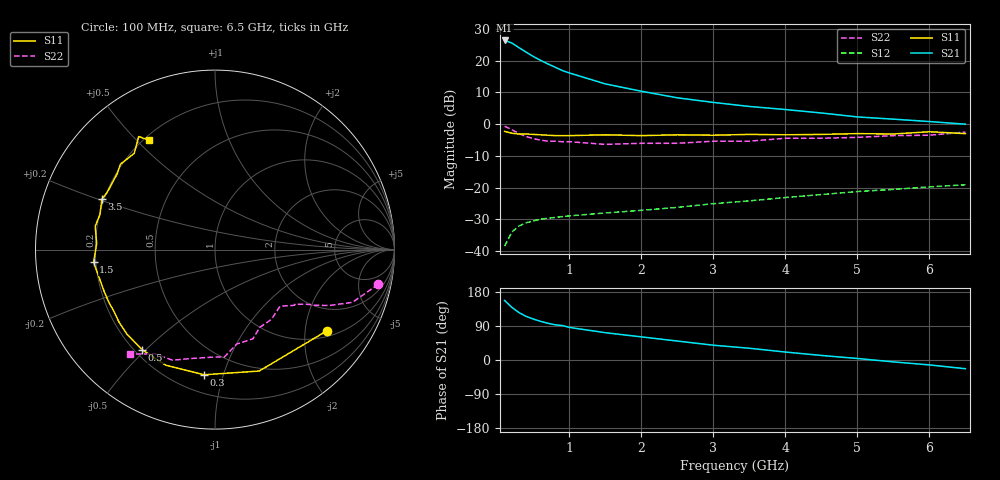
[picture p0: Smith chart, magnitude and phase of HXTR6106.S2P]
! HXTR-6106 Common Emitter
! Vce=15V  Ic=10mA
# ghz s ma r 50
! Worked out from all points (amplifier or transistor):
!   21 points, 100 MHz to 6.5 GHz, reference 50 ohm
!   highest |S21| = 26.4 dB at 100 MHz (marker M1)
!   |S21| within 3 dB of that: start of sweep to 351.1 MHz
!   unconditionally stable (mu >= 1): 1.454 GHz to 4.9 GHz
!   at 400 MHz: K = 0.38, MSG = 26.9 dB, |S12| = -31.1 dB
!   at 1.5 GHz: K = 1.03, MAG = 19.3 dB, |S12| = -28.0 dB
!   at 6.5 GHz: K = 0.54, MSG = 9.5 dB, |S12| = -19.1 dB
!   S11 on the Smith chart (normalised r, x): 100 MHz: 1.17, -2.61; 300 MHz: 0.32, -0.87; 500 MHz: 0.23, -0.49; 1.5 GHz: 0.19, -0.05; 3.5 GHz: 0.19, +0.21; 6.5 GHz: 0.22, +0.54
0.1  0.77 -36.0  20.8 157.0  0.012 67.0  0.93 -12.0
0.2  0.72 -70.0  19 139.0  0.02 55.0  0.82 -21.0
0.3  0.7 -95.0  16 125.0  0.025 46.0  0.71 -26.0
0.4  0.7 -113.0  13.6 115.0  0.028 41.0  0.64 -29.0
0.5  0.69 -126.0  11.6 108.0  0.03 37.0  0.59 -31.0
0.6  0.68 -136.0  10.1 102.0  0.032 36.0  0.56 -33.0
0.7  0.67 -143.0  8.9 97.0  0.033 35.0  0.54 -34.0
0.8  0.66 -149.0  7.9 93.0  0.034 35.0  0.54 -35.0
0.9  0.66 -154.0  7 91.0  0.035 34.0  0.53 -36.0
1  0.66 -159.0  6.4 86.0  0.036 35.0  0.53 -36.0
1.5  0.68 -174.0  4.3 72.0  0.04 36.0  0.48 -41.0
2  0.66 177.0  3.3 61.0  0.044 40.0  0.5 -51.0
2.5  0.68 169.0  2.6 50.0  0.049 42.0  0.5 -60.0
3  0.67 163.0  2.2 39.0  0.056 44.0  0.54 -67.0
3.5  0.69 156.0  1.9 31.0  0.062 46.0  0.54 -77.0
4  0.68 152.0  1.7 21.0  0.07 46.0  0.6 -85.0
4.5  0.69 142.0  1.5 12.0  0.078 47.0  0.6 -92.0
5  0.71 138.0  1.3 4.0  0.087 46.0  0.62 -102.0
5.5  0.7 130.0  1.2 -5.0  0.094 42.0  0.66 -111.0
6  0.76 124.0  1.1 -13.0  0.103 42.0  0.67 -120.0
6.5  0.71 121.0  1 -23.0  0.111 38.0  0.75 -129.0
